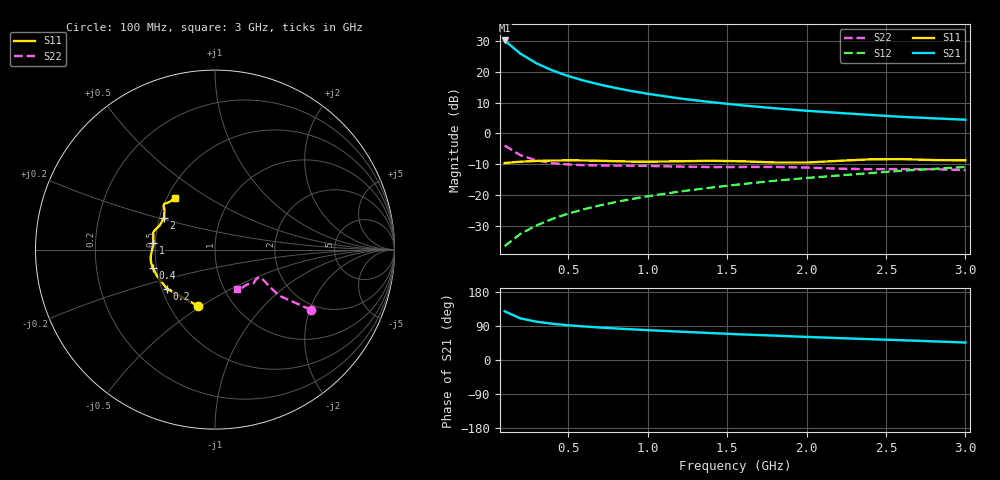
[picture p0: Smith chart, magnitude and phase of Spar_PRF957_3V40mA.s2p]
! Filename:  PRF957I.S2P  Version:  3.0
! NXP part #:  PRF957  Date:  Nov 1998
! Bias condition:  Vce=3V, Ic=40mA
#  MHz  S  MA  R 50
! Freq  S11  S21  S12  S22
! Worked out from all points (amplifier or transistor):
!   20 points, 100 MHz to 3 GHz, reference 50 ohm
!   highest |S21| = 30.2 dB at 100 MHz (marker M1)
!   |S21| within 3 dB of that: start of sweep to 169.4 MHz
!   unconditionally stable (mu >= 1): 387.5 MHz to end of sweep
!   at 400 MHz: K = 1.01, MAG = 23.7 dB, |S12| = -27.8 dB
!   at 1.2 GHz: K = 1.08, MAG = 13.4 dB, |S12| = -18.9 dB
!   at 3 GHz: K = 1.04, MAG = 6.5 dB, |S12| = -11.0 dB
!   S11 on the Smith chart (normalised r, x): 100 MHz: 0.69, -0.49; 200 MHz: 0.53, -0.26; 400 MHz: 0.48, -0.11; 1 GHz: 0.49, +0.04; 2 GHz: 0.53, +0.21; 3 GHz: 0.55, +0.37
100  0.3288 -106.3  32.2 128.5  0.01467 68.6  0.6322 -32.1
200  0.3455 -140.8  19.57 109.8  0.02327 70.0  0.4393 -35.7
300  0.3553 -155.5  13.72 101.1  0.03176 73.0  0.3629 -34.0
400  0.3611 -163.5  10.51 95.6  0.04059 75.1  0.3279 -32.5
500  0.3633 -168.5  8.51 91.7  0.04949 76.5  0.311 -31.9
600  0.3619 -172.2  7.157 88.5  0.05843 77.3  0.3032 -31.6
700  0.3574 -175.5  6.176 85.7  0.06739 77.9  0.3002 -31.6
800  0.3517 -178.8  5.436 83.2  0.07645 78.3  0.2991 -31.5
900  0.3471 177.7  4.85 80.9  0.08558 78.5  0.2976 -31.5
1000  0.3454 174.2  4.384 78.8  0.09474 78.6  0.2952 -31.6
1200  0.3508 168.1  3.688 74.9  0.1131 78.4  0.2877 -32.9
1400  0.3577 164.5  3.206 71.0  0.1312 77.9  0.2826 -36.0
1600  0.3503 161.4  2.833 67.4  0.15 77.4  0.2837 -39.1
1800  0.3357 156.1  2.548 64.3  0.1695 76.5  0.2842 -41.1
2000  0.3347 148.3  2.324 61.0  0.1879 75.9  0.2777 -42.9
2200  0.3564 142.0  2.148 57.8  0.2061 75.1  0.2667 -46.2
2400  0.3774 139.4  1.988 55.0  0.2255 74.0  0.2608 -51.0
2600  0.3805 137.8  1.849 52.2  0.2468 72.7  0.2621 -55.2
2800  0.3676 134.3  1.751 49.2  0.2642 72.0  0.2613 -57.9
3000  0.3631 127.6  1.663 46.2  0.2833 71.4  0.2528 -60.6
